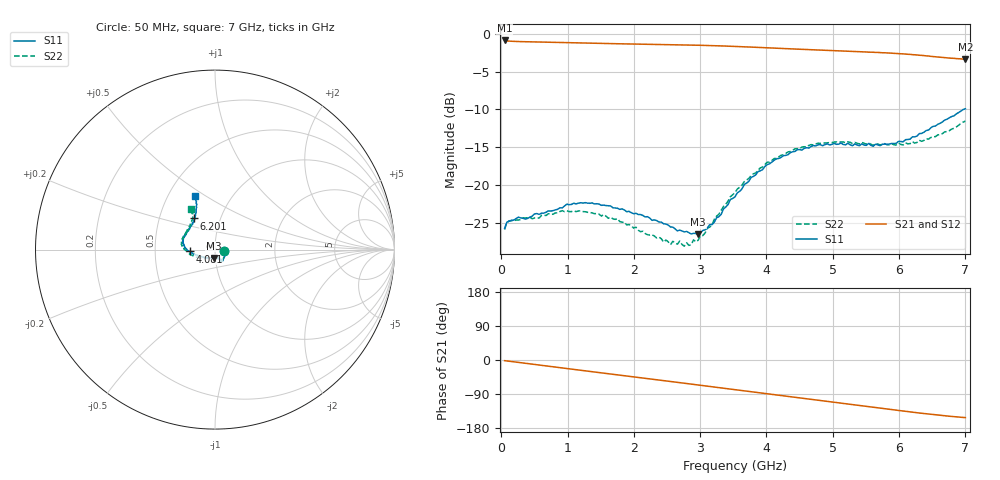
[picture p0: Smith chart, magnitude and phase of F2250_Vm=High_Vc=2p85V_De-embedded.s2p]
! Integrated Device Technology
! Corporate Headquarters
! 6024 Silver Creek Valley Road
! San Jose, CA 95138  USA
! Phone:  1-408-284-8200
! Toll Free:  1-800-223-1366
! Webpage:  http://www.idt.com/
! Timing and RF Division
! 515 Groton Road, Suite 102
! Westford, MA 01886-6024
! Device:  F2250
! Description: Voltage Variable RF Attenuator
! Frequency:  50.0 -  6000.00 MHz
! Package:  3x3 mm Thin QFN Plastic Package: 16 pin
! Ports:  2 RF, 3 DC
!  Pin  1  = GND
!  Pin  2  = NC
!  Pin  3  = RF1  = Port 1
!  Pin  4  = NC
!  Pin  5  = GND
!  Pin  6  = GND
!  Pin  7  = GND
!  Pin  8  = GND
!  Pin  9  = NC
!  Pin 10  = RF2  = Port 2
!  Pin 11  = NC
!  Pin 12  = GND
!  Pin 13  = GND
!  Pin 14  = VCNTRL
!  Pin 15  = VDD
!  Pin 16  = VMODE
! Vcntrl:  2.850 Volts
! Vmode:  +3.300 Volts
! Vdd:  +3.30  Volts
! Current:  1.314 mA
! Data:  The device was measured on a the F2250 evaluation board which has
!  individual transmission lines to the RF pins.  Data was collected
!  using a calibrated network analyzer.  The evaluation board was
!  de-embedded using a TRL calibration technique.
!  The reference plane is the edge of the package pin.
! Misc:  SN 10
!  Action Tracker AT0258
! Date Measured:  2014-11-26
! Date:  2015-10-15  MJV
! Note:
!  Integrated Device Technology supplies this data as a sample of measured
!  data at the package pin for this product.  Your particular data for this
!  product may vary.
!  Data was taken at 25 degrees C.
!  Integrated Device Technology reserves the right to change this data at anytime.
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# GHz S dB R 50
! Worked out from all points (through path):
!   201 points, 50 MHz to 7 GHz, reference 50 ohm
!   highest |S21| = -0.89 dB at 50 MHz (marker M1); lowest = -3.4 dB at 7 GHz (marker M2)
!   group delay of S21, straight-line fit = 61.1 ps
!   lowest |S11| = -26.5 dB at 2.969 GHz (marker M3), VSWR 1.10, Z = 49.1 - j4.62 ohm
!   |S11| at or under -10 dB: start of sweep to 6.967 GHz
!   |S22| runs from -28.0 to -11.5 dB; largest |S21 - S12| = 0.002
!   S11 on the Smith chart (normalised r, x): 50 MHz: 1.11, -0.02; 4.081 GHz: 0.75, -0.02; 6.201 GHz: 0.75, +0.27; 7 GHz: 0.68, +0.45
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0.05  -25.69 -10.8  -0.89 -1.8  -0.89 -1.8  -25.85 -11.0
0.1195  -24.75 -10.1  -0.99 -3.2  -0.98 -3.2  -24.69 -8.8
0.57125  -23.84 -31.4  -1.10 -13.3  -1.10 -13.3  -24.34 -31.4
0.91875  -22.99 -50.1  -1.17 -21.0  -1.17 -21.1  -23.35 -51.0
1.2315  -22.36 -57.9  -1.24 -27.9  -1.24 -27.9  -23.47 -61.5
1.75275  -23.04 -64.9  -1.33 -39.1  -1.33 -39.1  -24.42 -67.8
2.37825  -24.86 -64.5  -1.42 -52.8  -1.42 -52.8  -26.86 -66.7
2.552  -25.52 -69.5  -1.44 -56.7  -1.45 -56.7  -27.85 -73.1
2.691  -25.93 -77.5  -1.47 -59.8  -1.47 -59.8  -27.36 -80.8
2.7605  -26.17 -79.7  -1.48 -61.3  -1.48 -61.3  -28.04 -85.2
2.969  -26.49 -97.8  -1.52 -66.0  -1.52 -66.0  -27.27 -104.8
3.1775  -25.20 -120.8  -1.57 -70.7  -1.57 -70.7  -25.24 -126.7
3.525  -21.54 -152.7  -1.68 -78.5  -1.68 -78.6  -20.97 -148.7
3.76825  -18.96 -164.8  -1.77 -84.0  -1.77 -84.1  -18.70 -159.6
4.081  -16.95 -175.7  -1.90 -91.0  -1.90 -91.0  -16.72 -171.4
4.4285  -15.54 176.0  -2.03 -98.6  -2.03 -98.7  -15.19 178.7
4.7065  -14.76 169.1  -2.13 -104.8  -2.13 -104.8  -14.68 173.0
5.054  -14.60 160.9  -2.26 -112.5  -2.25 -112.5  -14.28 166.0
5.85325  -14.57 135.0  -2.56 -130.0  -2.56 -130.1  -14.67 147.3
6.20075  -13.62 123.6  -2.77 -137.7  -2.77 -137.8  -14.24 138.3
6.54825  -12.18 115.6  -3.04 -144.7  -3.04 -144.9  -13.58 126.9
7  -9.91 110.7  -3.36 -152.1  -3.37 -152.2  -11.54 120.7
